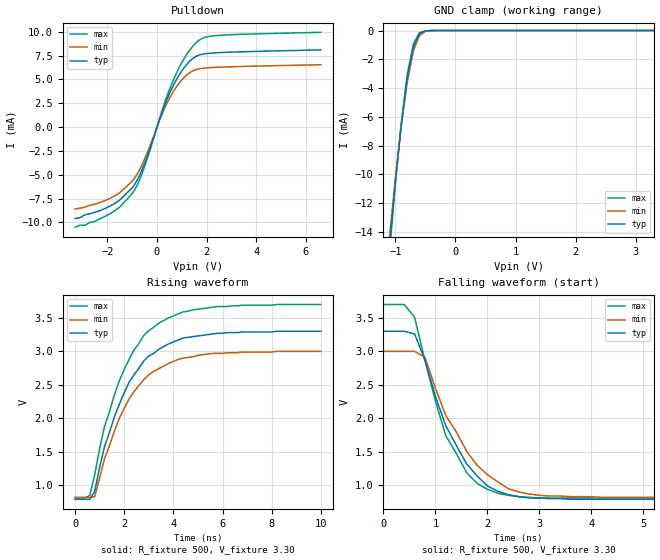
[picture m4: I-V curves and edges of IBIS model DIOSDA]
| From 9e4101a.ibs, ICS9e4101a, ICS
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|   Model DIOSDA
[Model]   DIOSDA
Model_type   I/O_open_drain
Polarity   Inverting
Enable   Active-High
Vinl =   0.80V
Vinh =   2.00V
C_comp   5.50pF   5.00pF   6.00pF
[Temperature Range]   27.00   70.00   0.000
[Voltage Range]   3.30V   3.00V   3.70V
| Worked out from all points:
|   slope of the pulldown table from 0 to 0.495 V, typ, clamps not added: 143 ohm
|   GND clamp passes 1 mA (typ) near -0.69 V on its own axis
|   rising waveform, R_fixture 500, V_fixture 3.30: 20-80 % time 1.67ns typ, 1.66ns min, 1.69ns max; typ from 0.79 V to 3.3 V
|   falling waveform, R_fixture 500, V_fixture 3.30: 20-80 % time 804ps typ, 912ps min, 744ps max; typ from 3.3 V to 0.79 V
[Pulldown]
| voltage   I(typ)   I(min)   I(max)
-3.3V     -9.6mA     -8.6mA     -10.5mA
-2.5V     -8.94mA    -8.09mA    -9.9mA
-1.9V     -8.3mA     -7.49mA    -9.1mA
-1.5V     -7.66mA    -6.89mA    -8.39mA
-1V       -6.37mA    -5.68mA    -6.99mA
-600mV    -4.47mA    -3.95mA    -4.87mA
200mV     1.54mA     1.34mA     1.71mA
700mV     4.58mA     3.89mA     5.18mA
1.2V      6.58mA     5.47mA     7.64mA
1.7V      7.57mA     6.12mA     9.13mA
2.6V      7.83mA     6.3mA      9.65mA
6.6V      8.11mA     6.55mA     9.95mA
[GND_clamp]
| voltage   I(typ)   I(min)   I(max)
-3.3V     -140mA     -130mA     -150mA
-1.1V     -15.08mA   -14.4mA    -15.5mA
-1V       -10.49mA   -10.23mA   -10.61mA
-900mV    -6.46mA    -6.53mA    -6.34mA
-800mV    -3.23mA    -3.51mA    -2.98mA
-700mV    -1.12mA    -1.4mA     -910uA
-600mV    -230uA     -360uA     -150uA
-500mV    -28.36uA   -59.14uA   -15.28uA
-400mV    -2.5uA     -7.33uA    -1.01uA
3.3V      150pA      520pA      120pA
[Ramp]
| variable   typ   min   max
dV/dt_r   1.50/2.03n   1.31/1.65n   1.74/1.65n
dV/dt_f   1.51/0.75n   1.31/0.85n   1.74/0.69n
R_load = 500
[Rising Waveform]
R_fixture = 500
V_fixture = 3.30
V_fixture_min = 3.00
V_fixture_max = 3.70
| time   V(typ)   V(min)   V(max)
0s        790mV      820mV      810mV
600ps     790mV      820mV      850mV
800ps     910mV      830mV      1.16V
1.2ns     1.58V      1.4V       1.88V
1.8ns     2.21V      2V         2.56V
2.2ns     2.54V      2.29V      2.88V
3ns       2.93V      2.65V      3.31V
3.8ns     3.11V      2.82V      3.5V
4.8ns     3.22V      2.92V      3.62V
10ns      3.3V       3V         3.7V
[Falling Waveform]
R_fixture = 500
V_fixture = 3.30
V_fixture_min = 3.00
V_fixture_max = 3.70
| time   V(typ)   V(min)   V(max)
0s        3.3V       3V         3.7V
400ps     3.3V       3V         3.7V
600ps     3.26V      3V         3.51V
800ps     2.87V      2.91V      2.86V
1.2ns     1.89V      2.04V      1.74V
1.6ns     1.32V      1.51V      1.19V
2.2ns     910mV      1.05V      880mV
2.6ns     830mV      900mV      830mV
3.2ns     800mV      840mV      810mV
10ns      790mV      820mV      810mV
